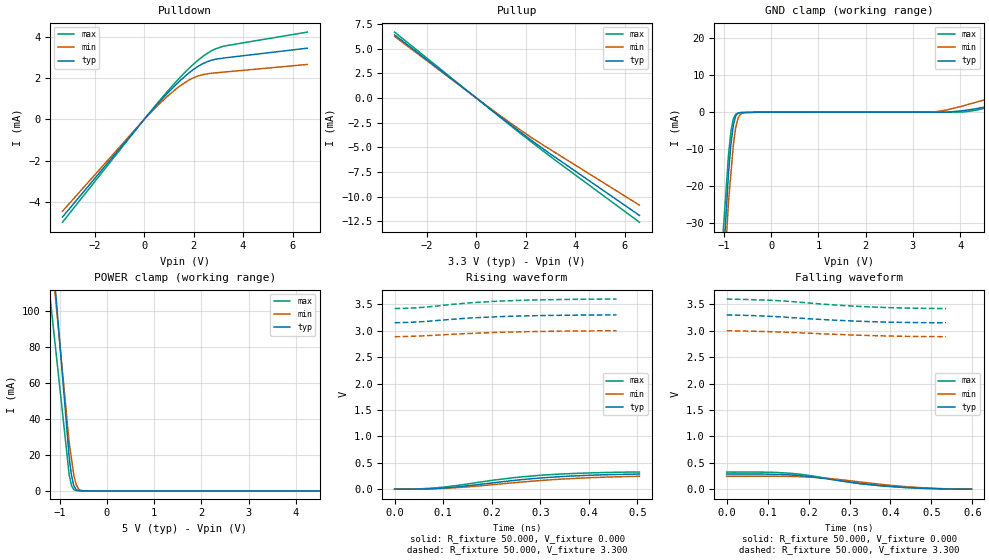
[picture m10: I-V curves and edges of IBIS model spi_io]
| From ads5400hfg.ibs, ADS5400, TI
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[Model]   spi_io
Model_type I/O
Vinl=8.000E-01
Vinh=2.000E+00
Vref=0.000E+00
Rref=1.000E+06
Cref=0.000E+00
Vmeas=1.650E+00
C_comp   4.600E-13   4.580E-13   4.660E-13
[Voltage Range]   3.300E+00   3.000E+00   3.600E+00
[POWER Clamp Reference]   5.000E+00   4.750E+00   5.250E+00
[GND Clamp Reference]   0.000E+00   0.000E+00   0.000E+00
[Pullup Reference]   3.300E+00   3.000E+00   3.600E+00
[Pulldown Reference]   0.000E+00   0.000E+00   0.000E+00
[Temperature Range]   25   85   -40
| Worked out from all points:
|   slope of the pulldown table from 0 to 0.495 V, typ, clamps not added: 728 ohm
|   slope of the pullup table from 0 to 0.495 V, typ, clamps not added: 508 ohm
|   GND clamp passes 1 mA (typ) near -0.75 V on its own axis
|   POWER clamp passes 1 mA (typ) near -0.66 V on its own axis
|   rising waveform, R_fixture 50.000, V_fixture 0.000: 20-80 % time 184ps typ, 195ps min, 171ps max; typ from 0 V to 0.286 V
|   falling waveform, R_fixture 50.000, V_fixture 0.000: 20-80 % time 179ps typ, 177ps min, 172ps max; typ from 0.286 V to 0 V
|   rising waveform, R_fixture 50.000, V_fixture 3.300: 20-80 % time 158ps typ, 177ps min, 152ps max; typ from 3.15 V to 3.3 V
|   falling waveform, R_fixture 50.000, V_fixture 3.300: 20-80 % time 207ps typ, 223ps min, 202ps max; typ from 3.3 V to 3.15 V
[GND Clamp]
-5V       -891mA     -895.3mA   -761.5mA
-900mV    -16.02mA   -23.84mA   -11.17mA
-850mV    -8.487mA   -16.32mA   -5.149mA
-800mV    -3.473mA   -8.801mA   -1.734mA
-750mV    -981.8uA   -4.107mA   -508.1uA
-700mV    -229.6uA   -1.54mA    -213.8uA
-650mV    -69.04uA   -575.8uA   -140.3uA
-275mV    -3.703uA   -7.898uA   -4.785uA
3.45V     1.359uA    109.2uA    949.1nA
4.2V      673.3uA    2.207mA    267.8uA
4.65V     1.669mA    3.816mA    1.469mA
10V       13.86mA    22.94mA    21.32mA
[POWER Clamp]
-5V       1.364A     1.193A     1.033A
-1.05V    98.7mA     96.26mA    69.93mA
-800mV    18.62mA    26.83mA    8.973mA
-750mV    8.359mA    17.66mA    2.895mA
-700mV    2.739mA    8.486mA    595.8uA
-650mV    661.8uA    3.314mA    157.1uA
-600mV    176.7uA    981.7uA    61.32uA
-550mV    85.04uA    242.8uA    54.11uA
-400mV    38.66uA    13.73uA    32.46uA
10V       0A         0A         0A
[Pullup]
-3.3V     6.391mA    6.233mA    6.673mA
500mV     -983.6uA   -937uA     -1.019mA
1.84V     -3.56mA    -3.343mA   -3.7mA
3.04V     -5.753mA   -5.302mA   -6.013mA
6.6V      -11.91mA   -10.87mA   -12.6mA
[Pulldown]
-3.3V     -4.715mA   -4.434mA   -4.966mA
160mV     225.6uA    203.7uA    239.7uA
600mV     821.3uA    732.7uA    876.6uA
1.3V      1.695mA    1.478mA    1.831mA
1.7V      2.133mA    1.82mA     2.33mA
1.98V     2.401mA    2.005mA    2.652mA
2.34V     2.676mA    2.155mA    3.014mA
2.54V     2.784mA    2.202mA    3.181mA
2.86V     2.901mA    2.248mA    3.396mA
3.2V      2.965mA    2.285mA    3.538mA
6.6V      3.443mA    2.656mA    4.22mA
[Rising Waveform]
R_fixture = 50.000
V_fixture = 0.000
V_fixture_min = 0.000
V_fixture_max = 0.000
|  time   V(typ)   V(min)   V(max)
0s        155.5uV    325.8uV    202.9uV
54ps      2.954mV    2.261mV    7.12mV
91ps      15.93mV    11.45mV    29.79mV
140ps     52.97mV    36.74mV    84.37mV
208ps     124.8mV    89.76mV    176.2mV
248ps     166.5mV    123mV      219.9mV
304ps     213.2mV    165.5mV    265.5mV
391ps     259.2mV    212mV      304.1mV
468ps     280.3mV    236.4mV    321.3mV
504ps     285.6mV    243.4mV    323.2mV
[Falling Waveform]
R_fixture = 50.000
V_fixture = 0.000
V_fixture_min = 0.000
V_fixture_max = 0.000
|  time   V(typ)   V(min)   V(max)
0s        285.6mV    243.4mV    323.2mV
121ps     281.3mV    243.7mV    316.3mV
167ps     263.5mV    238.9mV    292.2mV
204ps     236.1mV    227.8mV    256.6mV
251ps     188.9mV    201.9mV    195.7mV
314ps     118.2mV    148.2mV    116.1mV
386ps     60.31mV    83.88mV    56.97mV
476ps     19.14mV    28.28mV    16.41mV
556ps     1.192mV    1.958mV    423.9uV
598ps     155.5uV    325.8uV    202.9uV
[Rising Waveform]
R_fixture = 50.000
V_fixture = 3.300
V_fixture_min = 3.000
V_fixture_max = 3.600
|  time   V(typ)   V(min)   V(max)
0s        3.152V     2.887V     3.42V
21ps      3.157V     2.891V     3.424V
48ps      3.168V     2.899V     3.436V
60ps      3.174V     2.904V     3.444V
155ps     3.241V     2.949V     3.529V
189ps     3.257V     2.962V     3.548V
228ps     3.27V      2.973V     3.566V
275ps     3.283V     2.983V     3.58V
341ps     3.293V     2.993V     3.592V
457ps     3.3V       3V         3.6V
[Falling Waveform]
R_fixture = 50.000
V_fixture = 3.300
V_fixture_min = 3.000
V_fixture_max = 3.600
|  time   V(typ)   V(min)   V(max)
0s        3.3V       3V         3.6V
75ps      3.284V     2.989V     3.586V
123ps     3.266V     2.978V     3.571V
165ps     3.245V     2.966V     3.549V
236ps     3.212V     2.941V     3.503V
322ps     3.18V      2.916V     3.462V
355ps     3.172V     2.908V     3.45V
420ps     3.16V      2.897V     3.433V
469ps     3.154V     2.891V     3.426V
536ps     3.152V     2.887V     3.42V
[Ramp]
dV/dt_r   1.6701E-01/1.8302E-10   1.4147E-01/1.9428E-10   1.8896E-01/1.7150E-10
dV/dt_f   8.8777E-02/2.0512E-10   2.4000E+00/2.2325E-10   1.0776E-01/2.0125E-10
R_load = 50
